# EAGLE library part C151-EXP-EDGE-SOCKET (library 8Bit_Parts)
PIN HEADER
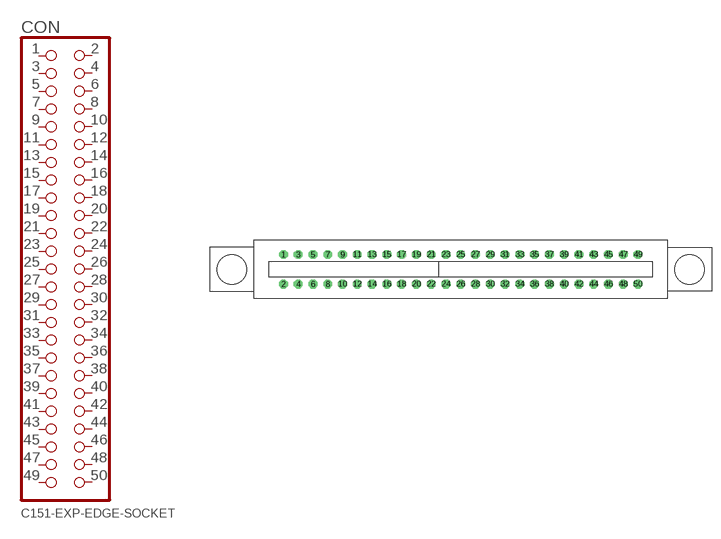
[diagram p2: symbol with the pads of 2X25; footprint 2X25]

Designator prefix CON

## C151-EXP-EDGE-SOCKET  [2X25]
1  1  pas
2  2  pas
3  3  pas
4  4  pas
5  5  pas
6  6  pas
7  7  pas
8  8  pas
9  9  pas
10  10  pas
11  11  pas
12  12  pas
13  13  pas
14  14  pas
15  15  pas
16  16  pas
17  17  pas
18  18  pas
19  19  pas
20  20  pas
21  21  pas
22  22  pas
23  23  pas
24  24  pas
25  25  pas
26  26  pas
27  27  pas
28  28  pas
29  29  pas
30  30  pas
31  31  pas
32  32  pas
33  33  pas
34  34  pas
35  35  pas
36  36  pas
37  37  pas
38  38  pas
39  39  pas
40  40  pas
41  41  pas
42  42  pas
43  43  pas
44  44  pas
45  45  pas
46  46  pas
47  47  pas
48  48  pas
49  49  pas
50  50  pas

## Footprint 2X25 (pad centres in mm)
PIN HEADER
drill 1.016 octagon: 1 -30.48,6.35; 2 -30.48,1.27; 3 -27.94,6.35; 4 -27.94,1.27; 5 -25.4,6.35; 6 -25.4,1.27; 7 -22.86,6.35; 8 -22.86,1.27; 9 -20.32,6.35; 10 -20.32,1.27; 11 -17.78,6.35; 12 -17.78,1.27; 13 -15.24,6.35; 14 -15.24,1.27; 15 -12.7,6.35; 16 -12.7,1.27; 17 -10.16,6.35; 18 -10.16,1.27; 19 -7.62,6.35; 20 -7.62,1.27; 21 -5.08,6.35; 22 -5.08,1.27; 23 -2.54,6.35; 24 -2.54,1.27; 25 0,6.35; 26 0,1.27; 27 2.54,6.35; 28 2.54,1.27; 29 5.08,6.35; 30 5.08,1.27; 31 7.62,6.35; 32 7.62,1.27; 33 10.16,6.35; 34 10.16,1.27; 35 12.7,6.35; 36 12.7,1.27; 37 15.24,6.35; 38 15.24,1.27; 39 17.78,6.35; 40 17.78,1.27; 41 20.32,6.35; 42 20.32,1.27; 43 22.86,6.35; 44 22.86,1.27; 45 25.4,6.35; 46 25.4,1.27; 47 27.94,6.35; 48 27.94,1.27; 49 30.48,6.35; 50 30.48,1.27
